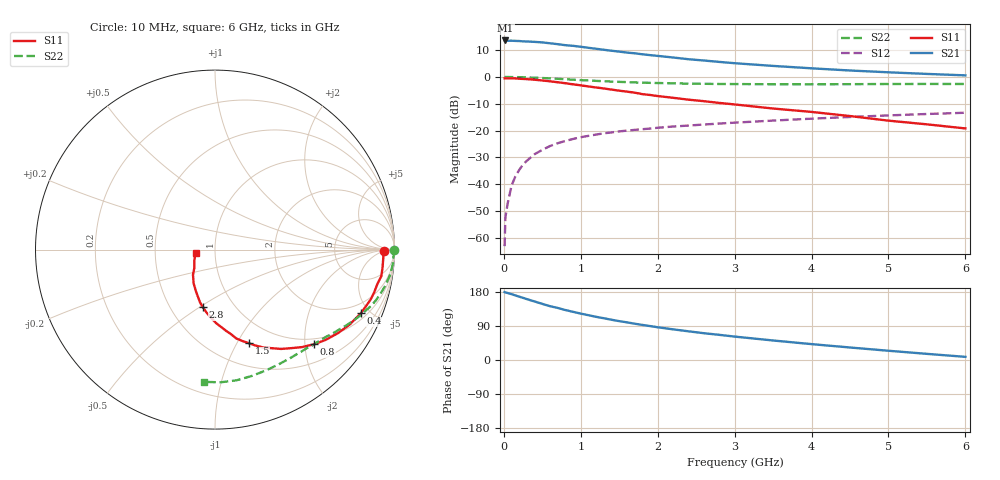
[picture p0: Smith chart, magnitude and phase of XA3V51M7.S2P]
! SIEMENS Discrete & RF Semiconductors
! BFY180
! Si NPN RF Bipolar Junction Transistor in MICRO-X
! VCE = 3.5 V  IC = 1.7 mA
! Common Emitter S-Parameters:  May  1997
# GHz  S  MA  R  50
!  f  S11  S21  S12  S22
! GHz  MAG  ANG  MAG  ANG  MAG  ANG  MAG  ANG
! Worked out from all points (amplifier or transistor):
!   36 points, 10 MHz to 6 GHz, reference 50 ohm
!   highest |S21| = 13.6 dB at 20 MHz (marker M1)
!   |S21| within 3 dB of that: start of sweep to 1.172 GHz
!   unconditionally stable (mu >= 1): 3.074 GHz to end of sweep
!   at 250 MHz: K = 0.11, MSG = 23.0 dB, |S12| = -32.7 dB
!   at 1.4 GHz: K = 0.63, MSG = 15.2 dB, |S12| = -20.7 dB
!   at 6 GHz: K = 1.07, MAG = 5.4 dB, |S12| = -13.4 dB
!   S11 on the Smith chart (normalised r, x): 10 MHz: 31, -5; 400 MHz: 1.33, -4.43; 800 MHz: 0.87, -2.21; 1.5 GHz: 0.74, -1.12; 2.8 GHz: 0.72, -0.52; 6 GHz: 0.80, -0.03
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0.01  0.9393 -0.6  4.725 179.1  0.0007 93.6  0.9946 -0.2
0.02  0.9393 -0.8  4.787 178.4  0.0024 85.8  0.9999 -0.7
0.05  0.9386 -3.0  4.716 176.8  0.0044 86.8  0.9961 -1.5
0.1  0.9388 -6.0  4.735 173.7  0.0094 85.8  0.9936 -3.2
0.15  0.9385 -9.1  4.693 170.4  0.014 84.0  0.9933 -4.7
0.25  0.9181 -15.1  4.603 164.0  0.0233 80.7  0.9867 -7.8
0.4  0.8875 -23.5  4.504 154.4  0.0363 75.4  0.969 -12.1
0.5  0.8587 -29.1  4.404 148.1  0.0437 71.3  0.954 -15.0
0.6  0.8287 -34.1  4.241 142.0  0.0515 68.4  0.9394 -17.6
0.8  0.7641 -43.6  3.907 131.8  0.064 62.8  0.9053 -22.1
0.9  0.7284 -48.2  3.8 127.1  0.0698 59.7  0.8888 -24.4
1.1  0.6645 -56.4  3.49 118.2  0.0797 55.5  0.8583 -28.2
1.2  0.6358 -59.8  3.351 113.9  0.0843 53.7  0.8446 -30.0
1.5  0.5547 -70.1  2.962 102.5  0.0966 49.1  0.8093 -34.8
1.8  0.4783 -79.4  2.645 92.6  0.1061 45.8  0.7819 -39.1
2.2  0.4085 -89.3  2.304 80.9  0.119 41.7  0.7609 -44.6
2.6  0.3532 -97.8  2.024 70.7  0.1297 38.6  0.7448 -49.7
2.8  0.3278 -101.8  1.906 66.4  0.1351 37.3  0.7393 -52.1
3.5  0.2577 -114.1  1.605 51.5  0.1536 32.4  0.7313 -60.8
4.5  0.1865 -131.1  1.318 33.0  0.1793 25.3  0.7331 -73.7
5.5  0.1307 -152.0  1.138 16.2  0.2038 17.6  0.7401 -87.7
6  0.1096 -169.4  1.07 8.3  0.215 13.6  0.7393 -94.6
